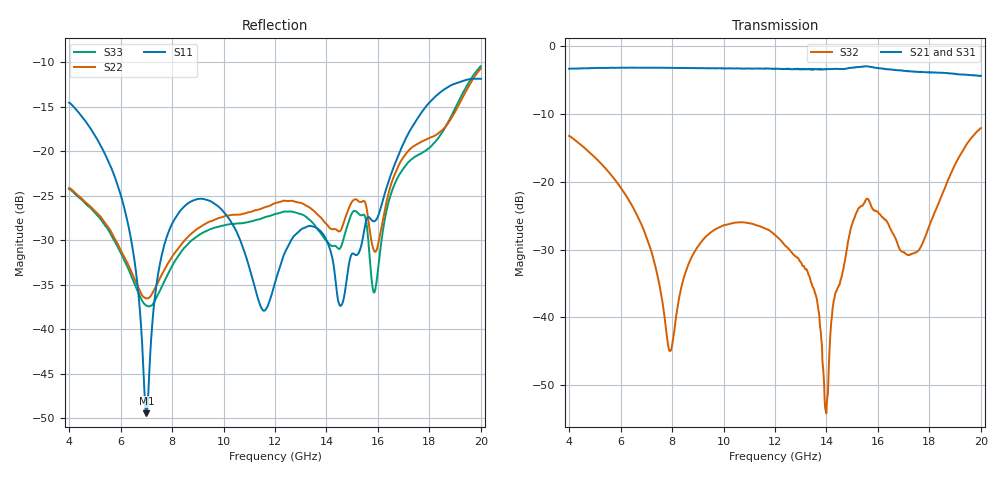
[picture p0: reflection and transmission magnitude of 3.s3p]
!The following data was pulled from an Agilent PNA
!This sNp file was generated from the data in the RF Test software
!NOTE:  Smoothing/Math/Corrections applied on any given trace ARE included in the data saved here
# MHz S dB R 50
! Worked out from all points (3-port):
!   1601 points, 4 GHz to 20 GHz, reference 50 ohm
!   strongest paths, dB at 4 GHz, 8 GHz, 12 GHz, 16 GHz, 20 GHz:
!     S21: -3.3, -3.2, -3.3, -3.2, -4.3
!     S31: -3.3, -3.2, -3.3, -3.2, -4.3
!     S32: -13.2, -44.2, -27.8, -24.4, -12.1
!   lowest |S11| = -49.4 dB at 7 GHz (marker M1), VSWR 1.01, Z = 50.1 - j0.328 ohm
!   |S11| at or under -10 dB: start of sweep to end of sweep
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4000  -14.53 90.4  -3.30 -108.6  -3.30 -109.0
      -3.29 -108.5  -24.12 -59.8  -13.22 -139.7
      -3.30 -108.9  -13.22 -139.7  -24.24 -59.7
6140  -26.34 33.8  -3.15 -170.4  -3.16 -171.1
      -3.15 -170.4  -31.89 -126.8  -21.60 163.0
      -3.15 -171.1  -21.59 163.0  -32.21 -130.5
7000  -49.45 -76.0  -3.15 163.9  -3.16 163.1
      -3.14 164.0  -36.52 -102.5  -28.11 142.8
      -3.17 163.2  -28.10 142.9  -37.33 -109.2
7910  -28.73 172.5  -3.15 136.4  -3.17 135.5
      -3.17 136.4  -32.28 -73.1  -44.88 -165.9
      -3.17 135.5  -44.94 -166.3  -33.39 -74.1
8490  -26.15 153.5  -3.18 118.6  -3.18 117.7
      -3.20 118.5  -30.02 -74.1  -33.71 -106.2
      -3.20 117.6  -33.71 -106.2  -30.81 -75.3
12000  -34.76 -91.4  -3.30 5.0  -3.32 3.7
       -3.31 5.3  -25.83 -90.3  -27.83 165.7
       -3.30 4.0  -27.83 165.7  -27.05 -92.9
13990  -29.91 134.6  -3.35 -64.9  -3.39 -66.2
       -3.40 -64.7  -28.14 -100.6  -54.31 42.6
       -3.40 -66.4  -54.16 42.5  -30.05 -102.8
15190  -31.64 -129.5  -3.08 -110.4  -3.05 -112.3
       -3.07 -110.4  -25.46 -88.3  -24.36 -127.0
       -3.04 -112.2  -24.36 -127.0  -26.84 -91.1
16830  -20.20 -37.1  -3.52 179.7  -3.51 177.8
       -3.55 179.9  -21.43 -71.1  -29.75 163.2
       -3.59 178.1  -29.79 163.1  -22.63 -71.6
20000  -11.85 160.7  -4.53 39.8  -4.50 37.5
       -4.34 39.2  -10.70 36.2  -12.03 159.5
       -4.34 37.0  -12.07 159.7  -10.43 33.4
